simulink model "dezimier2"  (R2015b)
settings: Solver=VariableStepAuto  StartTime=0.0  StopTime=10.0  RelTol=1e-3
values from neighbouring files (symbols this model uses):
  hTP = fir1(nord, 2*fp/fs)    [dezimier_2.m]    (also in dezimier_3.m; frac_delay_1.m = fir1(nord, fp*2); frac_delay_2.m = fir1(nord, fp*2); lagrange_3.m = fir1(40, 0.5))
  M = 5    [dezimier_1.m]    (also in dezimier_11.m; dezimier_2.m; dezimier_3.m; farrow_3.m)
  Ts = 1/fs    (= 5e-05)    [basisband_1.m]    (also in basisband_2.m = 5e-06; dezimier_1.m = 0.0005; dezimier_11.m = 0.0005; dezimier_2.m = 0.0005)
libraries: simulink x1, dspsigops x1

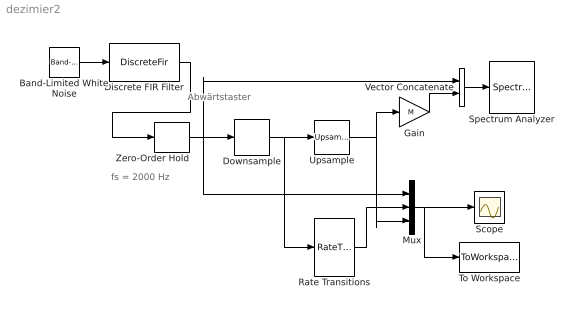
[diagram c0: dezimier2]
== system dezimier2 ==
  note: Abwärtstaster
  note: fs = 2000 Hz
  Band-Limited White Noise : simulink/Sources/Band-Limited White Noise  Cov=Ts/10  Ts=Ts  seed=[23341]
  Discrete FIR Filter : DiscreteFir  Coefficients=hTP  SampleTime=Ts
  Downsample : DownSample  N=M  RateOptions=Allow multirate processing
  Gain : Gain  Gain=M
  Mux : Mux  Inputs=3
  Rate Transitions : RateTransition
  Scope : Scope
  Spectrum Analyzer : SpectrumAnalyzer
  To Workspace : ToWorkspace  VariableName=y  SaveFormat=Timeseries  SampleTime=-1
  Upsample : dspsigops/Upsample  N=M  phase=0  RateOptions=Allow multirate processing  ic=0  mode=Unused parameter value
  Vector Concatenate : Concatenate  Mode=Multidimensional array  ConcatenateDimension=2
  Zero-Order Hold : ZeroOrderHold  SampleTime=Ts
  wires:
  Discrete FIR Filter/1 -> Zero-Order Hold/1
  Mux/1 -> To Workspace/1, Scope/1
  Zero-Order Hold/1 -> Vector Concatenate/1, Mux/1, Downsample/1
  Vector Concatenate/1 -> Spectrum Analyzer/1
  Downsample/1 -> Rate Transitions/1, Upsample/1
  Band-Limited White Noise/1 -> Discrete FIR Filter/1
  Upsample/1 -> Gain/1, Mux/3
  Rate Transitions/1 -> Mux/2
  Gain/1 -> Vector Concatenate/2
